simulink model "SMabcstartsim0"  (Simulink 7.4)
settings: Solver=ode45  StartTime=0.0  StopTime=10  MaxStep=2e-4  RelTol=1e-3
InitFcn:
  | smparamstartsim0
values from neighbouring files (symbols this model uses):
  Bm = 0.10    (= 0.1)    [IMabc2.m]    (also in imabcparam.m = 0.01; IMabcrun0.m = 0.01; IMabcrun1.m = 0.001; IMcur0.m = 1e-06)
  D = str2num(get(h,'string'))    [acttrcalc1.m]
  gam = 2*pi/3    (= 2.09439510239)    [IMabc2.m]    (also in IMabcf0.m; IMabcf1.m; imabcparam.m; IMabcrun0.m)
  H = 0.60    (= 0.6)    [IMabc2.m]    (also in IMcur0.m = 0.3; imdef0vec.m = 0.3; imdef1vec.m = 0.3; imdef2vec.m = 0.3)
  Lrr = [Lr   -Lm/2 -Lm/2    [IMabc2.m]    (also in IMabcf0.m = [Lr   -Lm1/2 -Lm1/2; IMabcf1.m = [Lr   -Lm1/2 -Lm1/2)
  Lss = [Ls   -Lm/2 -Lm/2    [IMabc2.m]    (also in IMabcf0.m = [Ls   -Lm1/2 -Lm1/2; IMabcf1.m = [Ls   -Lm1/2 -Lm1/2)
  Vm = Vll*sqrt(2/3)    [imabcparam.m]
  wo = 2*pi*freq0    [calc0.m]    (also in IMabc2.m = 376.991118431; imabcparam.m = 376.991118431; IMabcrun0.m = 376.991118431; IMabcrun1.m = 376.991118431)
undefined symbols (not defined in the file or in its folder): Laf, Lakd, Lakq, R1, R2, Row, TL1, TL2, vector

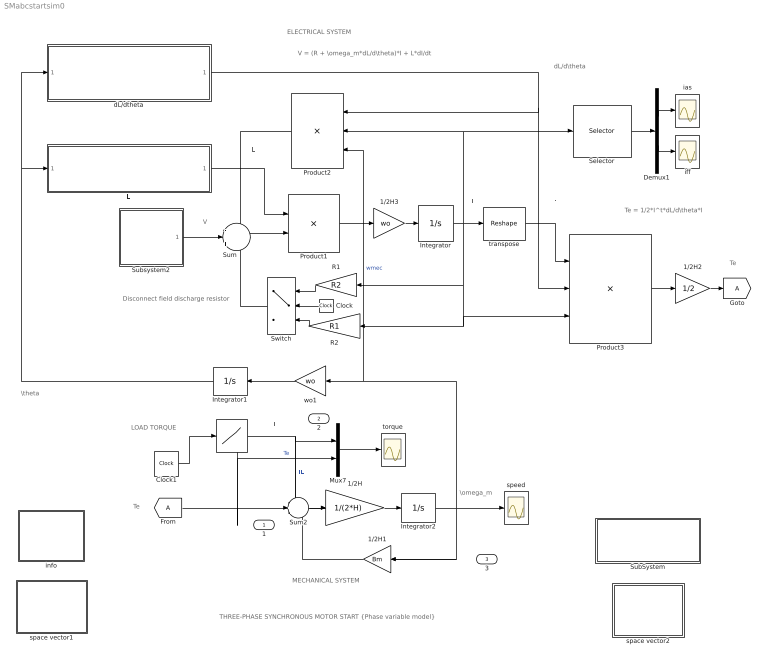
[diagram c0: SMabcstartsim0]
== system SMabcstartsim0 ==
  note: I
  note: I'
  note: MECHANICAL SYSTEM
  note: ELECTRICAL SYSTEM
  note: V
  note: THREE-PHASE SYNCHRONOUS MOTOR START {Phase variable model}
  note: L
  note: Te
  note: TL
  note: Te
  note: LOAD TORQUE
  note: Disconnect field discharge resistor
  note: dL/d\theta
  note: \omega_m
  note: \theta
  note: Te = 1/2*I^t*dL/d\theta*I
  note: V = (R + \omega_m*dL/d\theta)*I + L*dI/dt
  " " : Lookup  InputValues=[0 8 8 10 ]  Table="[TL1 TL1  TL2  TL2]"  OutDataType=sfix(16)  OutScaling=2^0
  1/2H : Gain  Gain=1/(2*H)  ParameterDataType=sfix(16)  ParameterScaling=2^0  OutDataType=sfix(16)  OutScaling=2^0
  1/2H1 : Gain  Gain=Bm  ParameterDataType=sfix(16)  ParameterScaling=2^0  OutDataType=sfix(16)  OutScaling=2^0
  1/2H2 : Gain  Gain=1/2  ParameterDataType=sfix(16)  ParameterScaling=2^0  OutDataType=sfix(16)  OutScaling=2^0
  1/2H3 : Gain  Gain=wo  ParameterDataType=sfix(16)  ParameterScaling=2^0  OutDataType=sfix(16)  OutScaling=2^0
  Clock : Clock
  Clock1 : Clock
  Demux1 : Demux  Outputs=2
  Integrator : Integrator  InitialCondition=[0 ;0 ;0; 0 ;0 ;0]
  Integrator1 : Integrator
  Integrator2 : Integrator
  L : Subsystem
  Mux7 : Mux  Inputs=2
  Product1 : Product  Inputs=/*  Multiplication=Matrix(*)  OutDataType=sfix(16)  OutScaling=2^0
  Product2 : Product  Inputs=***  Multiplication=Matrix(*)  OutDataType=sfix(16)  OutScaling=2^0
  Product3 : Product  Inputs=3  Multiplication=Matrix(*)  OutDataType=sfix(16)  OutScaling=2^0
  R1 : Gain  Gain=R2  Multiplication=Matrix(K*u)  ParameterDataType=sfix(16)  ParameterScaling=2^0  OutDataType=sfix(16)  OutScaling=2^0
  R2 : Gain  Gain=R1  Multiplication=Matrix(K*u)  ParameterDataType=sfix(16)  ParameterScaling=2^0  OutDataType=sfix(16)  OutScaling=2^0
  Selector : Selector  InputPortWidth=6  IndexOptions=Index vector (dialog)  Indices=[1 4]  OutputSizes=1
  SubSystem : Subsystem
  Subsystem2 : Subsystem
  Sum : Sum  Inputs=-|+|-  OutDataType=sfix(16)  OutScaling=2^0
  Sum2 : Sum  Inputs=-+-  OutDataType=sfix(16)  OutScaling=2^0
  Switch : Switch  Threshold=4
  dL/dtheta : Subsystem
  ias : Scope
  iff : Scope
  info : Subsystem
  space vector1 : Subsystem
  space vector2 : Subsystem
  speed : Scope
  torque : Scope
  transpose : Reshape  OutputDimensionality=Row vector (2-D)  OutputDimensions=[1,6]
  wo1 : Gain  Gain=wo  ParameterDataType=sfix(16)  ParameterScaling=2^0  OutDataType=sfix(16)  OutScaling=2^0
  1 : Outport
  2 : Outport  Port=2
  3 : Outport  Port=3
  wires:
  Product1/1 -> 1/2H3/1
  Sum/1 -> Product1/2
  transpose/1 -> Product3/1
  Product2/1 -> Sum/1
  dL/dtheta/1(dLdtheta) -> Product2/1, Product3/2
  Product3/1 -> 1/2H2/1
  Sum2/1 -> 1/2H/1
  1/2H/1 -> Integrator2/1
  1/2H1/1 -> Sum2/3
  Mux7/1 -> torque/1
  " "/1 -> Mux7/1, Sum2/1, 2/1  "TL"
  [A] -> Sum2/2, 1/1, Mux7/2  "Te"
  Integrator2/1 -> Product2/3, wo1/1, speed/1, 1/2H1/1, 3/1  "wmec"
  Subsystem2/1(V) -> Sum/2
  Integrator1/1 -> dL/dtheta/1(theta1), L/1(theta)
  Clock1/1 -> " "/1
  1/2H2/1 -> [A]
  L/1(L) -> Product1/1
  R2/1 -> Switch/3
  R1/1 -> Switch/1
  Clock/1 -> Switch/2
  Switch/1 -> Sum/3
  Integrator/1 -> transpose/1, Product2/2, Selector/1, Product3/3, R2/1, R1/1
  Selector/1 -> Demux1/1
  Demux1/2 -> iff/1
  Demux1/1 -> ias/1
  1/2H3/1 -> Integrator/1
  wo1/1 -> Integrator1/1

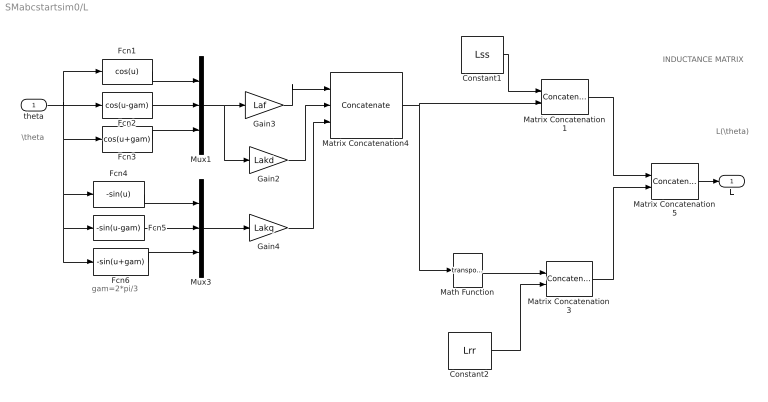
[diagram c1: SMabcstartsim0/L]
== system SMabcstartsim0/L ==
  note: INDUCTANCE MATRIX
  note: \theta
  note: gam=2*pi/3
  note: L(\theta)
  theta : Inport  OutDataType=sfix(16)  OutScaling=2^0
  Constant1 : Constant  Value=Lss  VectorParams1D=off  OutDataType=sfix(16)  OutScaling=2^0
  Constant2 : Constant  Value=Lrr  VectorParams1D=off  OutDataType=sfix(16)  OutScaling=2^0
  Fcn1 : Fcn  Expr=cos(u)
  Fcn2 : Fcn  Expr=cos(u-gam)
  Fcn3 : Fcn  Expr=cos(u+gam)
  Fcn4 : Fcn  Expr=-sin(u)
  Fcn5 : Fcn  Expr=-sin(u-gam)
  Fcn6 : Fcn  Expr=-sin(u+gam)
  Gain2 : Gain  Gain=Lakd  ParameterDataType=sfix(16)  ParameterScaling=2^0  OutDataType=sfix(16)  OutScaling=2^0
  Gain3 : Gain  Gain=Laf  ParameterDataType=sfix(16)  ParameterScaling=2^0  OutDataType=sfix(16)  OutScaling=2^0
  Gain4 : Gain  Gain=Lakq  ParameterDataType=sfix(16)  ParameterScaling=2^0  OutDataType=sfix(16)  OutScaling=2^0
  Math Function : Math  Operator=transpose
  Matrix Concatenation1 : Concatenate  Mode=Multidimensional array  ConcatenateDimension=2
  Matrix Concatenation3 : Concatenate  Mode=Multidimensional array  ConcatenateDimension=2
  Matrix Concatenation4 : Concatenate  NumInputs=3  Mode=Multidimensional array  ConcatenateDimension=2
  Matrix Concatenation5 : Concatenate  Mode=Multidimensional array
  Mux1 : Mux  Inputs=3
  Mux3 : Mux  Inputs=3
  L : Outport
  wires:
  Matrix Concatenation5/1 -> L/1
  Matrix Concatenation4/1 -> Matrix Concatenation1/2, Math Function/1
  Mux1/1 -> Gain3/1, Gain2/1
  Matrix Concatenation1/1 -> Matrix Concatenation5/1
  Constant1/1 -> Matrix Concatenation1/1
  Fcn3/1 -> Mux1/3
  Fcn2/1 -> Mux1/2
  Fcn1/1 -> Mux1/1
  theta/1 -> Fcn2/1, Fcn1/1, Fcn3/1, Fcn6/1, Fcn5/1, Fcn4/1
  Gain3/1 -> Matrix Concatenation4/1
  Gain2/1 -> Matrix Concatenation4/2
  Fcn5/1 -> Mux3/2
  Fcn4/1 -> Mux3/1
  Fcn6/1 -> Mux3/3
  Mux3/1 -> Gain4/1
  Gain4/1 -> Matrix Concatenation4/3
  Constant2/1 -> Matrix Concatenation3/2
  Matrix Concatenation3/1 -> Matrix Concatenation5/2
  Math Function/1 -> Matrix Concatenation3/1

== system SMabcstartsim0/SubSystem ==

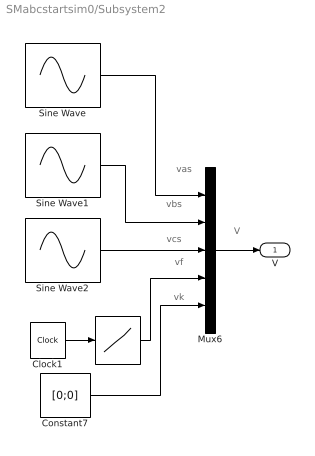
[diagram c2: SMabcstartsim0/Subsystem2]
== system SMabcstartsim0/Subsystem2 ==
  note: V
  note: vas
  note: vbs
  note: vcs
  note: vk
  note: vf
  " " : Lookup  InputValues=[0 4 4 10 ]  Table="[0  0  .02  0.02]"  OutDataType=sfix(16)  OutScaling=2^0
  Clock1 : Clock
  Constant7 : Constant  Value=[0;0]  VectorParams1D=off  OutDataType=sfix(16)  OutScaling=2^0
  Mux6 : Mux  Inputs=5
  Sine Wave : Sin  Amplitude=Vm  Bias=0  Frequency=wo  Phase=pi/2  Samples=10  SampleTime=0
  Sine Wave1 : Sin  Amplitude=Vm  Bias=0  Frequency=wo  Phase=pi/2-gam  Samples=10  SampleTime=0
  Sine Wave2 : Sin  Amplitude=Vm  Bias=0  Frequency=wo  Phase=pi/2+gam  Samples=10  SampleTime=0
  V : Outport
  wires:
  Mux6/1 -> V/1
  Sine Wave2/1 -> Mux6/3
  Sine Wave1/1 -> Mux6/2
  Sine Wave/1 -> Mux6/1
  Constant7/1 -> Mux6/5
  Clock1/1 -> " "/1
  " "/1 -> Mux6/4

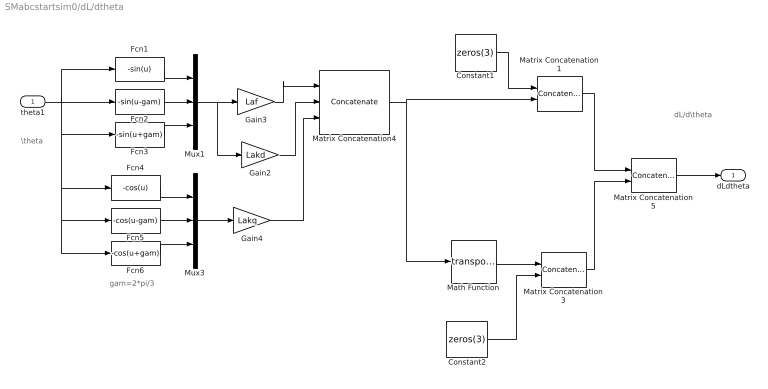
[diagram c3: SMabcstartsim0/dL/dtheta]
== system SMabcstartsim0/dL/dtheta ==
  note: dL/d\theta
  note: gam=2*pi/3
  note: \theta
  theta1 : Inport  OutDataType=sfix(16)  OutScaling=2^0
  Constant1 : Constant  Value=zeros(3)  VectorParams1D=off  OutDataType=sfix(16)  OutScaling=2^0
  Constant2 : Constant  Value=zeros(3)  VectorParams1D=off  OutDataType=sfix(16)  OutScaling=2^0
  Fcn1 : Fcn  Expr=-sin(u)
  Fcn2 : Fcn  Expr=-sin(u-gam)
  Fcn3 : Fcn  Expr=-sin(u+gam)
  Fcn4 : Fcn  Expr=-cos(u)
  Fcn5 : Fcn  Expr=-cos(u-gam)
  Fcn6 : Fcn  Expr=-cos(u+gam)
  Gain2 : Gain  Gain=Lakd  ParameterDataType=sfix(16)  ParameterScaling=2^0  OutDataType=sfix(16)  OutScaling=2^0
  Gain3 : Gain  Gain=Laf  ParameterDataType=sfix(16)  ParameterScaling=2^0  OutDataType=sfix(16)  OutScaling=2^0
  Gain4 : Gain  Gain=Lakq  ParameterDataType=sfix(16)  ParameterScaling=2^0  OutDataType=sfix(16)  OutScaling=2^0
  Math Function : Math  Operator=transpose
  Matrix Concatenation1 : Concatenate  Mode=Multidimensional array  ConcatenateDimension=2
  Matrix Concatenation3 : Concatenate  Mode=Multidimensional array  ConcatenateDimension=2
  Matrix Concatenation4 : Concatenate  NumInputs=3  Mode=Multidimensional array  ConcatenateDimension=2
  Matrix Concatenation5 : Concatenate  Mode=Multidimensional array
  Mux1 : Mux  Inputs=3
  Mux3 : Mux  Inputs=3
  dLdtheta : Outport
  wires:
  Matrix Concatenation5/1 -> dLdtheta/1
  Matrix Concatenation4/1 -> Matrix Concatenation1/2, Math Function/1
  Mux1/1 -> Gain3/1, Gain2/1
  Matrix Concatenation1/1 -> Matrix Concatenation5/1
  Constant1/1 -> Matrix Concatenation1/1
  Fcn3/1 -> Mux1/3
  Fcn2/1 -> Mux1/2
  Fcn1/1 -> Mux1/1
  theta1/1 -> Fcn2/1, Fcn1/1, Fcn3/1, Fcn6/1, Fcn5/1, Fcn4/1
  Gain3/1 -> Matrix Concatenation4/1
  Gain2/1 -> Matrix Concatenation4/2
  Fcn5/1 -> Mux3/2
  Fcn4/1 -> Mux3/1
  Fcn6/1 -> Mux3/3
  Mux3/1 -> Gain4/1
  Gain4/1 -> Matrix Concatenation4/3
  Constant2/1 -> Matrix Concatenation3/2
  Matrix Concatenation3/1 -> Matrix Concatenation5/2
  Math Function/1 -> Matrix Concatenation3/1

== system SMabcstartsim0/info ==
  note: START OF A SYNCHRONOUS MOTOR (Phase variable model) [pu]
  note: A cylindrical rotor synchronous motor is started from stanstill at rated voltage with the dc field circuit shorted across an external field discharge resistor. When synchronous is almost attained, the discharge resistor is removed and a dc voltage is applied to the field circuit so that the motor runs at synchronous speed. A load is then suddenly applied. The dynamic equations are expressed in matrix form in terms the phase variables, namely the stator currents ias, ibs, ics; the rotor field current iff; the d-axis and q-axis damper currents idk and iqk; the anglar speed wm; and the displacement angle theta between stator as-axis and rotor direct axis. Torque, speed and current responses are plotted. A Matlab script file for the identical system operation is given in the file >.

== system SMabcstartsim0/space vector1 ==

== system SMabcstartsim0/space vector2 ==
